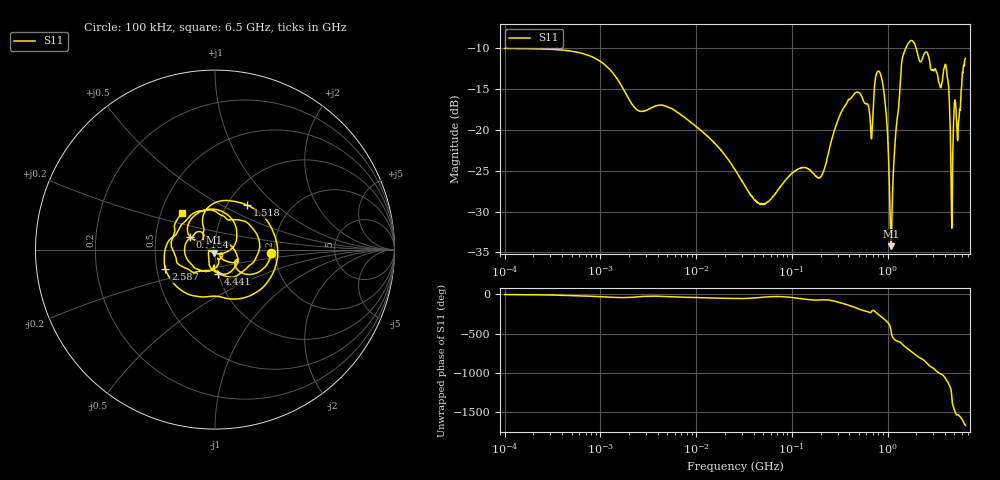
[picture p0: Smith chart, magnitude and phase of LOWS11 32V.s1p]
!Keysight Technologies,E5080B,MY59100498,A.17.05.10
!Date: Wednesday, August 30, 2023 18:49:34
!Correction: S11(C  1-Port  )
!S1P File: Measurement: S11:Log Frequency Sweep
# Hz S  dB  R 50
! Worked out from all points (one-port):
!   1601 points, 100 kHz to 6.5 GHz, reference 50 ohm
!   lowest |S11| = -34.2 dB at 1.089 GHz (marker M1), VSWR 1.04, Z = 49.2 - j1.76 ohm
!   |S11| at or under -10 dB: start of sweep to 1.553 GHz; 1.981 GHz to end of sweep
!   S11 on the Smith chart (normalised r, x): 100 kHz: 1.91, -0.07; 718.4 MHz: 0.75, +0.11; 1.518 GHz: 1.23, +0.67; 2.587 GHz: 0.56, -0.13; 4.441 GHz: 1.00, -0.28; 6.5 GHz: 0.64, +0.28
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100000  -10.07 -3.2
399589.6  -10.28 -12.7
1596718  -14.29 -41.4
2487396  -17.66 -32.0
6380321  -17.88 -34.5
2.54951e7  -24.88 -53.9
4.888947e7  -29.12 -37.8
1.018758e8  -25.25 -41.9
2.008454e8  -25.75 -71.2
4.070849e8  -16.24 -146.6
6.702952e8  -20.51 129.6
7.183677e8  -15.98 152.8
7.860529e8  -12.91 111.8
8.904243e8  -14.39 58.6
9.675956e8  -18.07 20.4
1.088507e9  -34.23 -112.8
1.330654e9  -15.91 115.3
1.517814e9  -10.30 54.1
1.626669e9  -9.53 25.9
2.002356e9  -10.19 -61.2
2.587259e9  -10.54 -158.4
3.274269e9  -13.03 97.7
4.115103e9  -12.64 -10.9
4.440884e9  -17.32 -81.9
4.759378e9  -26.50 47.6
5.065506e9  -16.38 -53.8
5.777982e9  -16.99 -122.6
6.5e9  -11.29 132.0
